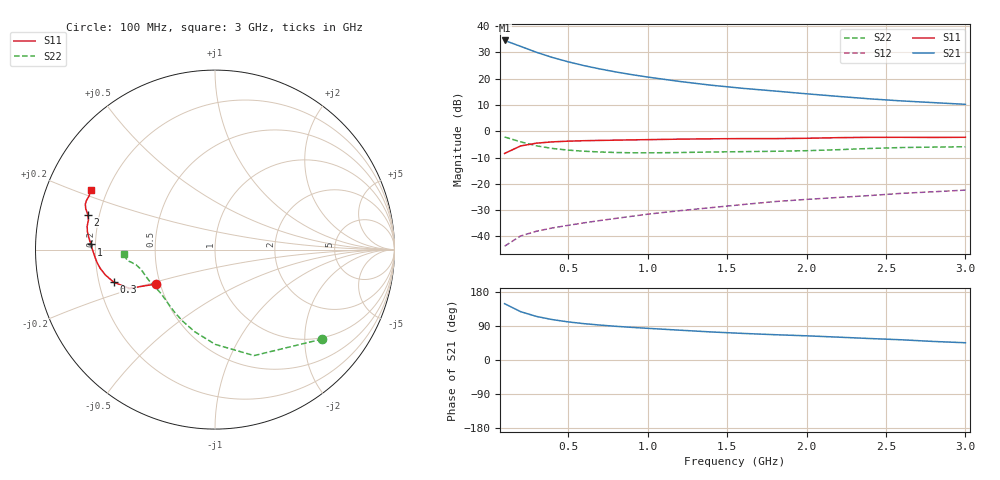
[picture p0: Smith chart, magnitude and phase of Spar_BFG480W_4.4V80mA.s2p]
! Filename: 4_480BFG480.001
! Title: BFG480W
! Bias: Vce=4.4V; Ic=80mA
! Company: NXP Semiconductors NL
! User: Quality&Reliability T&D
! Measure time: 10 Nov 1999 / 12:06:37
#  MHz  S  MA  R 50
! Freq  S11  S21  S12  S22  :
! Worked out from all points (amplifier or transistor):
!   20 points, 100 MHz to 3 GHz, reference 50 ohm
!   highest |S21| = 34.5 dB at 100 MHz (marker M1)
!   |S21| within 3 dB of that: start of sweep to 234.2 MHz
!   unconditionally stable (mu >= 1): 799.3 MHz to end of sweep
!   at 400 MHz: K = 0.75, MSG = 32.4 dB, |S12| = -36.8 dB
!   at 1.2 GHz: K = 1.07, MAG = 23.0 dB, |S12| = -30.2 dB
!   at 3 GHz: K = 1.05, MAG = 15.0 dB, |S12| = -22.4 dB
!   S11 on the Smith chart (normalised r, x): 100 MHz: 0.48, -0.21; 300 MHz: 0.26, -0.15; 1 GHz: 0.18, +0.02; 2 GHz: 0.16, +0.13; 3 GHz: 0.14, +0.23
100  0.378 -149.6  53.13 148.6  0.006539 68.0  0.7783 -39.8
200  0.5248 -155.7  41.11 127.7  0.0102 59.1  0.6293 -69.8
300  0.5932 -162.2  31.71 115.0  0.01256 57.4  0.5283 -89.8
400  0.6278 -167.1  25.29 106.6  0.0145 58.3  0.4709 -104.0
500  0.6479 -170.7  20.88 100.6  0.01627 60.1  0.4374 -114.3
600  0.6607 -173.7  17.66 95.9  0.01814 62.2  0.4168 -122.2
700  0.6694 -176.2  15.27 92.1  0.02007 64.4  0.4032 -128.3
800  0.6767 -178.4  13.4 88.9  0.02204 66.2  0.3942 -133.4
900  0.6851 179.5  11.91 86.2  0.02418 68.3  0.3895 -137.8
1000  0.692 177.6  10.71 83.6  0.02648 69.5  0.3881 -141.8
1200  0.7071 174.4  8.846 78.7  0.03085 71.4  0.3936 -148.2
1400  0.7181 172.0  7.493 74.0  0.03531 72.7  0.4029 -153.0
1600  0.7241 169.6  6.536 70.2  0.04042 73.7  0.409 -156.7
1800  0.7239 166.9  5.812 66.8  0.04601 74.5  0.416 -160.5
2000  0.7345 164.7  5.145 63.8  0.05063 75.5  0.4266 -165.0
2200  0.7551 162.5  4.594 60.3  0.05512 75.3  0.4461 -168.8
2400  0.7656 160.7  4.121 56.6  0.05994 75.0  0.4707 -171.3
2600  0.7666 159.1  3.768 53.3  0.06605 74.5  0.4902 -172.8
2800  0.7623 156.8  3.496 48.9  0.07075 73.1  0.4994 -174.6
3000  0.7673 154.1  3.247 45.5  0.07609 72.5  0.507 -177.5
